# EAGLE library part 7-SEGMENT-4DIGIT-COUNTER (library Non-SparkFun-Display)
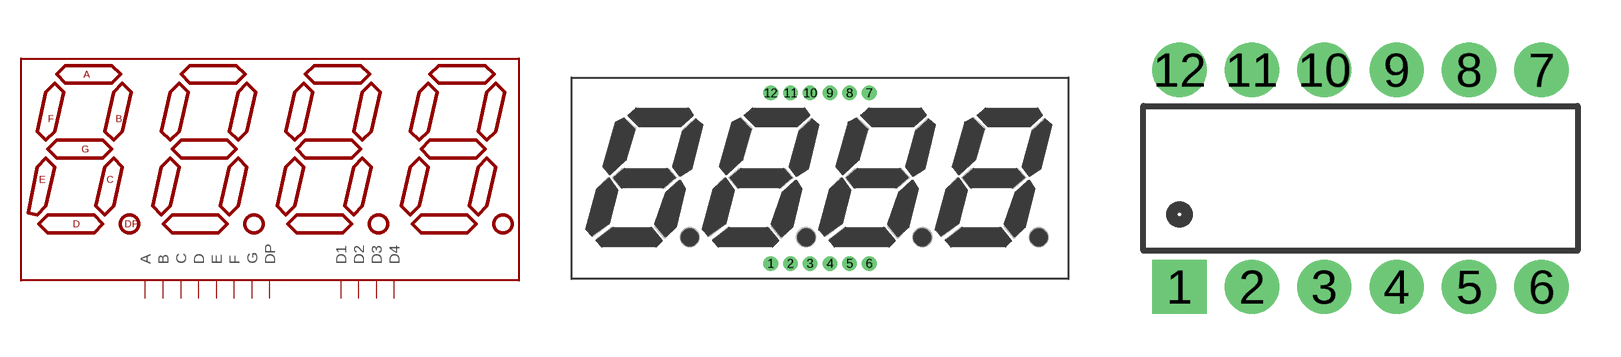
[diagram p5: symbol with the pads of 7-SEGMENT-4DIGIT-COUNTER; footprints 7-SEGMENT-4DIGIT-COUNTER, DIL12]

Designator prefix DISP

## 7-SEGMENT-4DIGIT-COUNTERPTH  [7-SEGMENT-4DIGIT-COUNTER]
1  E
2  D
3  DP
4  C
5  G
6  D4
7  B
8  D3
9  D2
10  F
11  A
12  D1

## 7-SEGMENT-4DIGIT-COUNTER-HP-BUBBLE (STOREFRONT: COM-12710)  [DIL12]
1  D1
2  E
3  C
4  D3
5  DP
6  D4
7  G
8  D
9  F
10  D2
11  B
12  A

## Footprint 7-SEGMENT-4DIGIT-COUNTER (pad centres in mm)
drill 0.9 pad 1.88: 1 -6.35,-10.998; 2 -3.81,-10.998; 3 -1.27,-10.998; 4 1.27,-10.998; 5 3.81,-10.998; 6 6.35,-10.998; 7 6.35,10.998; 8 3.81,10.998; 9 1.27,10.998; 10 -1.27,10.998; 11 -3.81,10.998; 12 -6.35,10.998

## Footprint DIL12 (pad centres in mm)
drill 0.864 pad 1.905 square: 1 -6.35,-3.81
drill 0.864 pad 1.905: 2 -3.81,-3.81; 3 -1.27,-3.81; 4 1.27,-3.81; 5 3.81,-3.81; 6 6.35,-3.81; 7 6.35,3.81; 8 3.81,3.81; 9 1.27,3.81; 10 -1.27,3.81; 11 -3.81,3.81; 12 -6.35,3.81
